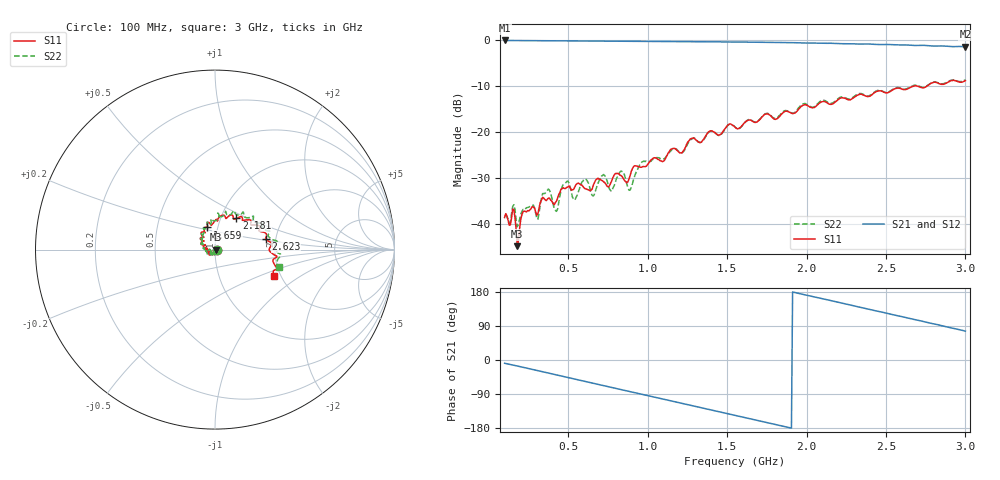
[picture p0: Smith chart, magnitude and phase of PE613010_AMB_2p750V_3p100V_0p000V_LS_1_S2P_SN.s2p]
!Agilent Technologies,N5230A,MY45001685,A.07.50.67
!Agilent N5230A: A.07.50.67
!Date: Monday, March 06, 2017 15:09:20
!Correction: S11(Full 2 Port(1,2))
!S21(Full 2 Port(1,2))
!S12(Full 2 Port(1,2))
!S22(Full 2 Port(1,2))
!S2P File: Measurements: S11, S21, S12, S22:
# Hz S  dB  R 50
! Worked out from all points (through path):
!   401 points, 100 MHz to 3 GHz, reference 50 ohm
!   highest |S21| = -0.15 dB at 100 MHz (marker M1); lowest = -1.5 dB at 3 GHz (marker M2)
!   group delay of S21, straight-line fit = 264 ps
!   lowest |S11| = -44.7 dB at 179.8 MHz (marker M3), VSWR 1.01, Z = 50.6 - j0.126 ohm
!   |S11| at or under -10 dB: start of sweep to 2.678 GHz; 2.694 GHz to 2.76 GHz (66.31 MHz wide, 2.43 % of centre)
!   |S22| runs from -40.5 to -8.7 dB; largest |S21 - S12| = 0.0025
!   S11 on the Smith chart (normalised r, x): 100 MHz: 1.02, -0.01; 1.659 GHz: 0.89, +0.22; 2.181 GHz: 1.19, +0.43; 2.623 GHz: 1.77, +0.22; 3 GHz: 1.85, -0.63
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1e8  -38.50 -12.5  -0.15 -8.6  -0.15 -8.6  -38.16 -11.7
1.7975e8  -44.71 -12.3  -0.17 -15.9  -0.17 -15.9  -40.50 -2.3
2.2325e8  -37.10 -46.1  -0.18 -19.9  -0.18 -20.0  -36.88 -48.7
3.03e8  -38.03 -50.1  -0.19 -27.5  -0.20 -27.5  -38.79 -54.5
3.6825e8  -34.57 -92.2  -0.21 -33.8  -0.20 -33.9  -32.61 -70.5
4.2625e8  -34.95 -70.4  -0.22 -39.3  -0.22 -39.3  -37.17 -80.3
4.77e8  -32.22 -114.5  -0.23 -44.2  -0.23 -44.2  -31.21 -93.8
5.4225e8  -31.85 -90.5  -0.24 -50.4  -0.23 -50.4  -34.73 -111.5
5.8575e8  -31.48 -120.4  -0.25 -54.6  -0.25 -54.6  -30.90 -108.9
7.235e8  -30.78 -146.4  -0.27 -67.7  -0.27 -67.7  -29.19 -117.0
7.7425e8  -30.54 -124.4  -0.28 -72.5  -0.28 -72.5  -32.83 -142.9
8.395e8  -29.60 -163.3  -0.29 -78.6  -0.30 -78.7  -28.53 -131.6
8.9025e8  -29.37 -134.4  -0.30 -83.5  -0.30 -83.5  -32.53 -166.3
9.6275e8  -27.61 -179.1  -0.32 -90.4  -0.32 -90.4  -26.52 -153.3
1.0715e9  -25.98 170.1  -0.34 -100.6  -0.34 -100.7  -25.56 -168.3
1.55e9  -18.91 121.4  -0.48 -146.0  -0.48 -146.0  -18.91 131.1
1.65875e9  -17.62 109.9  -0.52 -156.3  -0.53 -156.3  -17.55 118.3
2.03575e9  -14.72 70.5  -0.70 167.9  -0.69 167.8  -14.63 81.0
2.18075e9  -13.49 55.5  -0.79 154.0  -0.79 154.0  -13.30 65.4
2.5215e9  -11.30 21.8  -1.04 121.6  -1.03 121.6  -11.21 33.0
2.623e9  -10.79 11.4  -1.12 112.1  -1.11 112.0  -10.70 24.6
3e9  -8.85 -24.1  -1.52 76.2  -1.51 76.1  -8.67 -15.2
